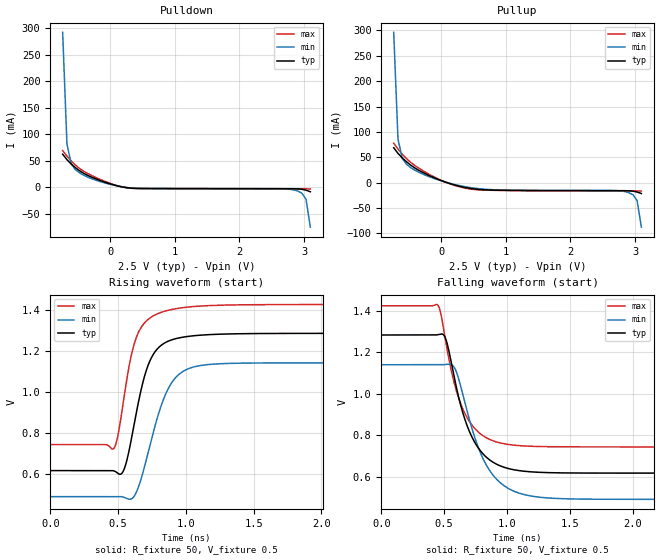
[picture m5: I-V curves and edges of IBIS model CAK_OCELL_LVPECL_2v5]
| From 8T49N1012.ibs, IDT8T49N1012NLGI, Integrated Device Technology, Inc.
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[Model] CAK_OCELL_LVPECL_2v5
Model_type   Output_ECL
Polarity   Non-Inverting
|   typ   min   max
C_comp   2pF   1.5pF   2.5pF
Vmeas = 0.923V
Rref = 50
Cref = 0
Vref = 0.5V
|   typ   min   max
[Voltage range]   2.5V   2.375V   2.625V
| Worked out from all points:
|   rising waveform, R_fixture 50, V_fixture 0.5: 20-80 % time 143ps typ, 177ps min, 127ps max; typ from 0.617 V to 1.28 V
|   falling waveform, R_fixture 50, V_fixture 0.5: 20-80 % time 202ps typ, 230ps min, 185ps max; typ from 1.28 V to 0.617 V
[Pulldown]
|Voltage   I (typ)   I (min)   I (max)
|Note, modeling breaks down at 250mA and above.  This is well beyond the functional   |
|operating range of the device.  Should this scenario occur, catastrophic failure and   |
|possible damage to the device and/or board is of higher concern than the I-V curve   |
|behavior.  The IBIS checker will flag currents in excess of 10A with warnings.  Lines   |
|with currents in excess of 0.35 A have been commented out.  The points still remain|
|available to the user if the user desires to use them.   |
|-2.20000e+00   2.53979e+01   2.10445e+01   3.04163e+01
|-1.90000e+00   1.96676e+01   1.67470e+01   2.30953e+01
|-1.60000e+00   1.39413e+01   1.24539e+01   1.57782e+01
|-1.30000e+00   8.21910e+00   8.16513e+00   8.46566e+00
|-1.00000e+00   2.50124e+00   3.88008e+00   1.15812e+00
|-9.99000e-01   2.48218e+00   3.86580e+00   1.13377e+00
|-9.32920e-01   1.22326e+00   2.92238e+00   1.66933e-01
|-8.66839e-01   2.54612e-01   1.97902e+00   9.11671e-02
|-8.00759e-01   8.49863e-02   1.03530e+00   8.00439e-02
-734.7mV  62.72mA    292.3mA    69.64mA
-668.6mV  52.4mA     82.35mA    59.12mA
-602.5mV  44.16mA    44.31mA    49.9mA
-536.4mV  37.15mA    33.4mA     42.05mA
-404.3mV  26.27mA    22.72mA    30.17mA
-140mV    12.38mA    10.48mA    14.4mA
124.4mV   2.639mA    2.54mA     2.794mA
322.6mV   -1.339mA   -1.009mA   -1.552mA
2.834V    -2.48mA    -4.344mA   -2.481mA
2.966V    -3.41mA    -10.72mA   -2.501mA
3.032V    -5.167mA   -22.22mA   -2.569mA
3.098V    -8.134mA   -74.82mA   -2.967mA
| 3.16407e+00   -1.22235e-02   -3.63034e-01   -4.39466e-03
| 3.23015e+00   -1.74780e-02   -9.07683e-01   -7.44621e-03
| 3.29623e+00   -2.66642e-02   -1.45780e+00   -1.20519e-02
| 3.36231e+00   -7.73349e-02   -2.00815e+00   -1.78304e-02
| 3.42839e+00   -5.10375e-01   -2.55868e+00   -2.39960e-02
| 3.49447e+00   -1.24402e+00   -3.10934e+00   -3.07890e-02
| 3.56055e+00   -1.97787e+00   -3.66011e+00   -6.28241e-02
| 3.62663e+00   -2.71193e+00   -4.21097e+00   -5.43092e-01
| 3.69271e+00   -3.44621e+00   -4.76193e+00   -1.48075e+00
| 3.75879e+00   -4.18069e+00   -5.31296e+00   -2.41855e+00
| 3.82487e+00   -4.91534e+00   -5.86408e+00   -3.35644e+00
| 3.89095e+00   -5.65013e+00   -6.41526e+00   -4.29442e+00
| 3.95703e+00   -6.38505e+00   -6.96652e+00   -5.23249e+00
| 4.02311e+00   -7.12006e+00   -7.51784e+00   -6.17069e+00
| 4.08920e+00   -7.85517e+00   -8.06923e+00   -7.10908e+00
| 4.15528e+00   -8.59035e+00   -8.62067e+00   -8.04767e+00
| 4.22136e+00   -9.32559e+00   -9.17217e+00   -8.98643e+00
| 4.28744e+00   -1.00609e+01   -9.72372e+00   -9.92532e+00
| 4.35352e+00   -1.07963e+01   -1.02753e+01   -1.08643e+01
| 4.41960e+00   -1.15317e+01   -1.08270e+01   -1.18033e+01
| 4.48568e+00   -1.22671e+01   -1.13787e+01   -1.27425e+01
| 4.55176e+00   -1.30026e+01   -1.19304e+01   -1.36816e+01
| 4.61784e+00   -1.37381e+01   -1.24822e+01   -1.46208e+01
| 4.68392e+00   -1.44737e+01   -1.30340e+01   -1.55600e+01
| 4.75000e+00   -1.52093e+01   -1.35859e+01   -1.64993e+01
| 4.75100e+00   -1.52204e+01   -1.35942e+01   -1.65135e+01
| 4.80080e+00   -1.57748e+01   -1.40102e+01   -1.72213e+01
| 4.85060e+00   -1.63292e+01   -1.44261e+01   -1.79292e+01
| 4.90040e+00   -1.68836e+01   -1.48421e+01   -1.86371e+01
| 4.95020e+00   -1.74380e+01   -1.52580e+01   -1.93450e+01
| 5.00000e+00   -1.79924e+01   -1.56740e+01   -2.00529e+01
[Pullup]
|Voltage   I (typ)   I (min)   I (max)
|Note, modeling breaks down at 250mA and above.  This is well beyond the functional   |
|operating range of the device.  Should this scenario occur, catastrophic failure and   |
|possible damage to the device and/or board is of higher concern than the I-V curve   |
|behavior.  The IBIS checker will flag currents in excess of 10A with warnings.  Lines   |
|with currents in excess of 0.35 A have been commented out.  The points still remain|
|available to the user if the user desires to use them.   |
|-2.20000e+00   2.54263e+01   2.10725e+01   3.04445e+01
|-1.90000e+00   1.96905e+01   1.67704e+01   2.31215e+01
|-1.60000e+00   1.39601e+01   1.24715e+01   1.58009e+01
|-1.30000e+00   8.23393e+00   8.17715e+00   8.48375e+00
|-1.00000e+00   2.51142e+00   3.88778e+00   1.17086e+00
|-9.99000e-01   2.49235e+00   3.87348e+00   1.14649e+00
|-9.32920e-01   1.23231e+00   2.92912e+00   1.78403e-01
|-8.66839e-01   2.62541e-01   1.98481e+00   1.01359e-01
|-8.00759e-01   9.17903e-02   1.04016e+00   8.89398e-02
-734.7mV  68.58mA    296.4mA    77.42mA
-668.6mV  57.55mA    85.91mA    66.01mA
-602.5mV  48.62mA    47.36mA    55.93mA
-536.4mV  40.89mA    35.93mA    47.16mA
-338.2mV  23.53mA    19.72mA    27.68mA
-73.87mV  7.576mA    6.44mA     8.848mA
454.8mV   -11.67mA   -10.05mA   -12.95mA
2.702V    -16.07mA   -15.9mA    -16.43mA
2.9V      -16.31mA   -19.81mA   -16.45mA
2.966V    -17.02mA   -23.95mA   -16.47mA
3.032V    -18.76mA   -35.45mA   -16.53mA
3.098V    -21.7mA    -88.06mA   -16.91mA
| 3.16407e+00   -2.57645e-02   -3.76288e-01   -1.83101e-02
| 3.23015e+00   -3.10025e-02   -9.20950e-01   -2.13305e-02
| 3.29623e+00   -4.01768e-02   -1.47108e+00   -2.59087e-02
| 3.36231e+00   -9.08409e-02   -2.02144e+00   -3.16663e-02
| 3.42839e+00   -5.23878e-01   -2.57197e+00   -3.78177e-02
| 3.49447e+00   -1.25752e+00   -3.12264e+00   -4.46027e-02
| 3.56055e+00   -1.99138e+00   -3.67341e+00   -7.66308e-02
| 3.62663e+00   -2.72546e+00   -4.22428e+00   -5.56891e-01
| 3.69271e+00   -3.45975e+00   -4.77524e+00   -1.49454e+00
| 3.75879e+00   -4.19425e+00   -5.32628e+00   -2.43231e+00
| 3.82487e+00   -4.92892e+00   -5.87740e+00   -3.37016e+00
| 3.89095e+00   -5.66373e+00   -6.42859e+00   -4.30806e+00
| 3.95703e+00   -6.39866e+00   -6.97985e+00   -5.24603e+00
| 4.02311e+00   -7.13368e+00   -7.53117e+00   -6.18421e+00
| 4.08920e+00   -7.86879e+00   -8.08256e+00   -7.12265e+00
| 4.15528e+00   -8.60398e+00   -8.63401e+00   -8.06132e+00
| 4.22136e+00   -9.33923e+00   -9.18551e+00   -9.00014e+00
| 4.28744e+00   -1.00745e+01   -9.73707e+00   -9.93908e+00
| 4.35352e+00   -1.08099e+01   -1.02887e+01   -1.08781e+01
| 4.41960e+00   -1.15453e+01   -1.08403e+01   -1.18172e+01
| 4.48568e+00   -1.22808e+01   -1.13920e+01   -1.27563e+01
| 4.55176e+00   -1.30163e+01   -1.19438e+01   -1.36955e+01
| 4.61784e+00   -1.37518e+01   -1.24956e+01   -1.46347e+01
| 4.68392e+00   -1.44874e+01   -1.30474e+01   -1.55739e+01
| 4.75000e+00   -1.52230e+01   -1.35993e+01   -1.65132e+01
| 4.75100e+00   -1.52341e+01   -1.36076e+01   -1.65274e+01
| 4.80080e+00   -1.57885e+01   -1.40236e+01   -1.72353e+01
| 4.85060e+00   -1.63429e+01   -1.44395e+01   -1.79432e+01
| 4.90040e+00   -1.68973e+01   -1.48555e+01   -1.86511e+01
| 4.95020e+00   -1.74518e+01   -1.52715e+01   -1.93590e+01
| 5.00000e+00   -1.80062e+01   -1.56875e+01   -2.00669e+01
[Ramp]
|   typ   min   max
dV/dt_r   0.411/0.144n   0.398/0.179n   0.422/0.128n
dV/dt_f   0.403/0.201n   0.392/0.23n   0.412/0.185n
R_load =   50.0000
[Rising Waveform]
R_fixture = 50
V_fixture = 0.5   | VCC_typ - 2V
V_fixture_max = 0.625   | VCC_max - 2V
V_fixture_min = 0.375   | VCC_min - 2V
C_fixture = 0.0p
| Time   typ   min   max
0s        616.8mV    490.1mV    743.4mV
462.2ps   616.4mV    490.1mV    721.3mV
528.9ps   604.3mV    489.5mV    906.8mV
591.1ps   746.5mV    477.3mV    1.158V
648.9ps   946mV      534.3mV    1.287V
737.8ps   1.155V     747.1mV    1.361V
862.2ps   1.244V     1.006V     1.396V
986.7ps   1.267V     1.103V     1.41V
1.209ns   1.28V      1.135V     1.421V
4ns       1.285V     1.141V     1.425V
[Falling Waveform]
R_fixture = 50
V_fixture = 0.5   | VCC_typ - 2V
V_fixture_max = 0.625   | VCC_max - 2V
V_fixture_min = 0.375   | VCC_min - 2V
C_fixture = 0.0p
| Time   typ   min   max
0s        1.284V     1.14V      1.425V
448.9ps   1.285V     1.14V      1.429V
511.1ps   1.268V     1.142V     1.258V
568.9ps   1.115V     1.137V     1.08V
640ps     926.7mV    1.018V     939.4mV
715.6ps   798.6mV    844.7mV    853.7mV
813.3ps   707.2mV    682.1mV    795.9mV
924.4ps   657.8mV    583.1mV    766mV
1.382ns   618.3mV    494.7mV    744.1mV
4ns       616.8mV    490.1mV    743.4mV
